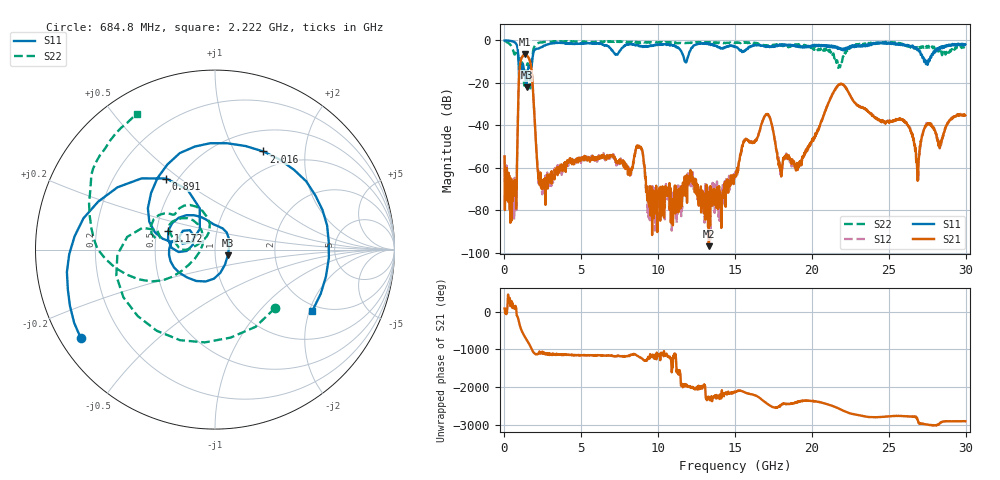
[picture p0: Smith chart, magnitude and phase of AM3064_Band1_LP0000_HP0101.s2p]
# Hz S DB R 50.0
!freq dBS11 angS11 dBS21 angS21 dBS12 angS12 dBS22 angS22
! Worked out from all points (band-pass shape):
!   1600 points, 10 MHz to 29.98 GHz, reference 50 ohm
!   highest |S21| = -6.63 dB at 1.322 GHz (marker M1); lowest = -97.0 dB at 13.3 GHz (marker M2)
!   |S21| within 3 dB of the highest: 1.056 GHz to 1.652 GHz (596.8 MHz wide, 44.1 % of centre)
!   lowest |S11| = -22.1 dB at 1.435 GHz (marker M3), VSWR 1.17, Z = 57.6 - j3.56 ohm
!   |S11| at or under -10 dB: 916.7 MHz to 1.798 GHz (881.1 MHz wide, 64.9 % of centre); 11.74 GHz to 11.84 GHz (103.4 MHz wide, 0.877 % of centre); 27.39171 GHz to 27.46104 GHz (69.33 MHz wide, 0.253 % of centre)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
!   |S22| runs from -22.6 to -0.2 dB; largest |S21 - S12| = 0.0046
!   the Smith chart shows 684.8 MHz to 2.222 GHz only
!   S11 on the Smith chart (normalised r, x): 684.8 MHz: 0.06, -0.30; 891 MHz: 0.43, +0.45; 1.172 GHz: 0.58, +0.13; 2.016 GHz: 0.76, +1.31; 2.222 GHz: 1.82, -2.10
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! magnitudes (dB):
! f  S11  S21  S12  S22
! 10 MHz  -0.1  -54.8  -54.1  -0.2
! 684.8 MHz  -1.0  -68.3  -70.0  -6.6
! 891 MHz  -6.4  -30.5  -30.5  -7.5
! 1.172 GHz  -11.0  -7.6  -7.5  -10.9
! 1.322 GHz  -17.0  -6.6  -6.6  -19.5
! 1.435 GHz  -22.1  -6.9  -6.9  -12.7
! 2.016 GHz  -4.3  -43.9  -43.6  -2.1
! 2.222 GHz  -3.9  -64.4  -67.2  -1.2
! 5.015 GHz  -1.3  -55.5  -55.7  -0.8
! 8.763 GHz  -2.8  -49.7  -50.0  -1.0
! 9.382 GHz  -2.7  -76.5  -79.5  -0.8
! 10 GHz  -2.0  -72.0  -77.9  -0.9
! 13.3 GHz  -1.8  -97.0  -95.7  -1.2
! 15 GHz  -3.0  -64.3  -64.2  -1.3
! 17.03 GHz  -3.1  -34.8  -34.9  -2.7
! 17.95 GHz  -2.2  -61.4  -62.7  -1.9
! 19.99 GHz  -2.9  -47.9  -48.1  -3.4
! 21.83 GHz  -3.8  -20.7  -20.5  -12.7
! 25 GHz  -1.0  -38.4  -38.0  -1.1
! 26.87 GHz  -4.4  -66.2  -63.5  -3.2
! 27.49 GHz  -9.9  -39.3  -39.8  -3.1
! 29.98 GHz  -1.9  -35.3  -35.2  -3.2
